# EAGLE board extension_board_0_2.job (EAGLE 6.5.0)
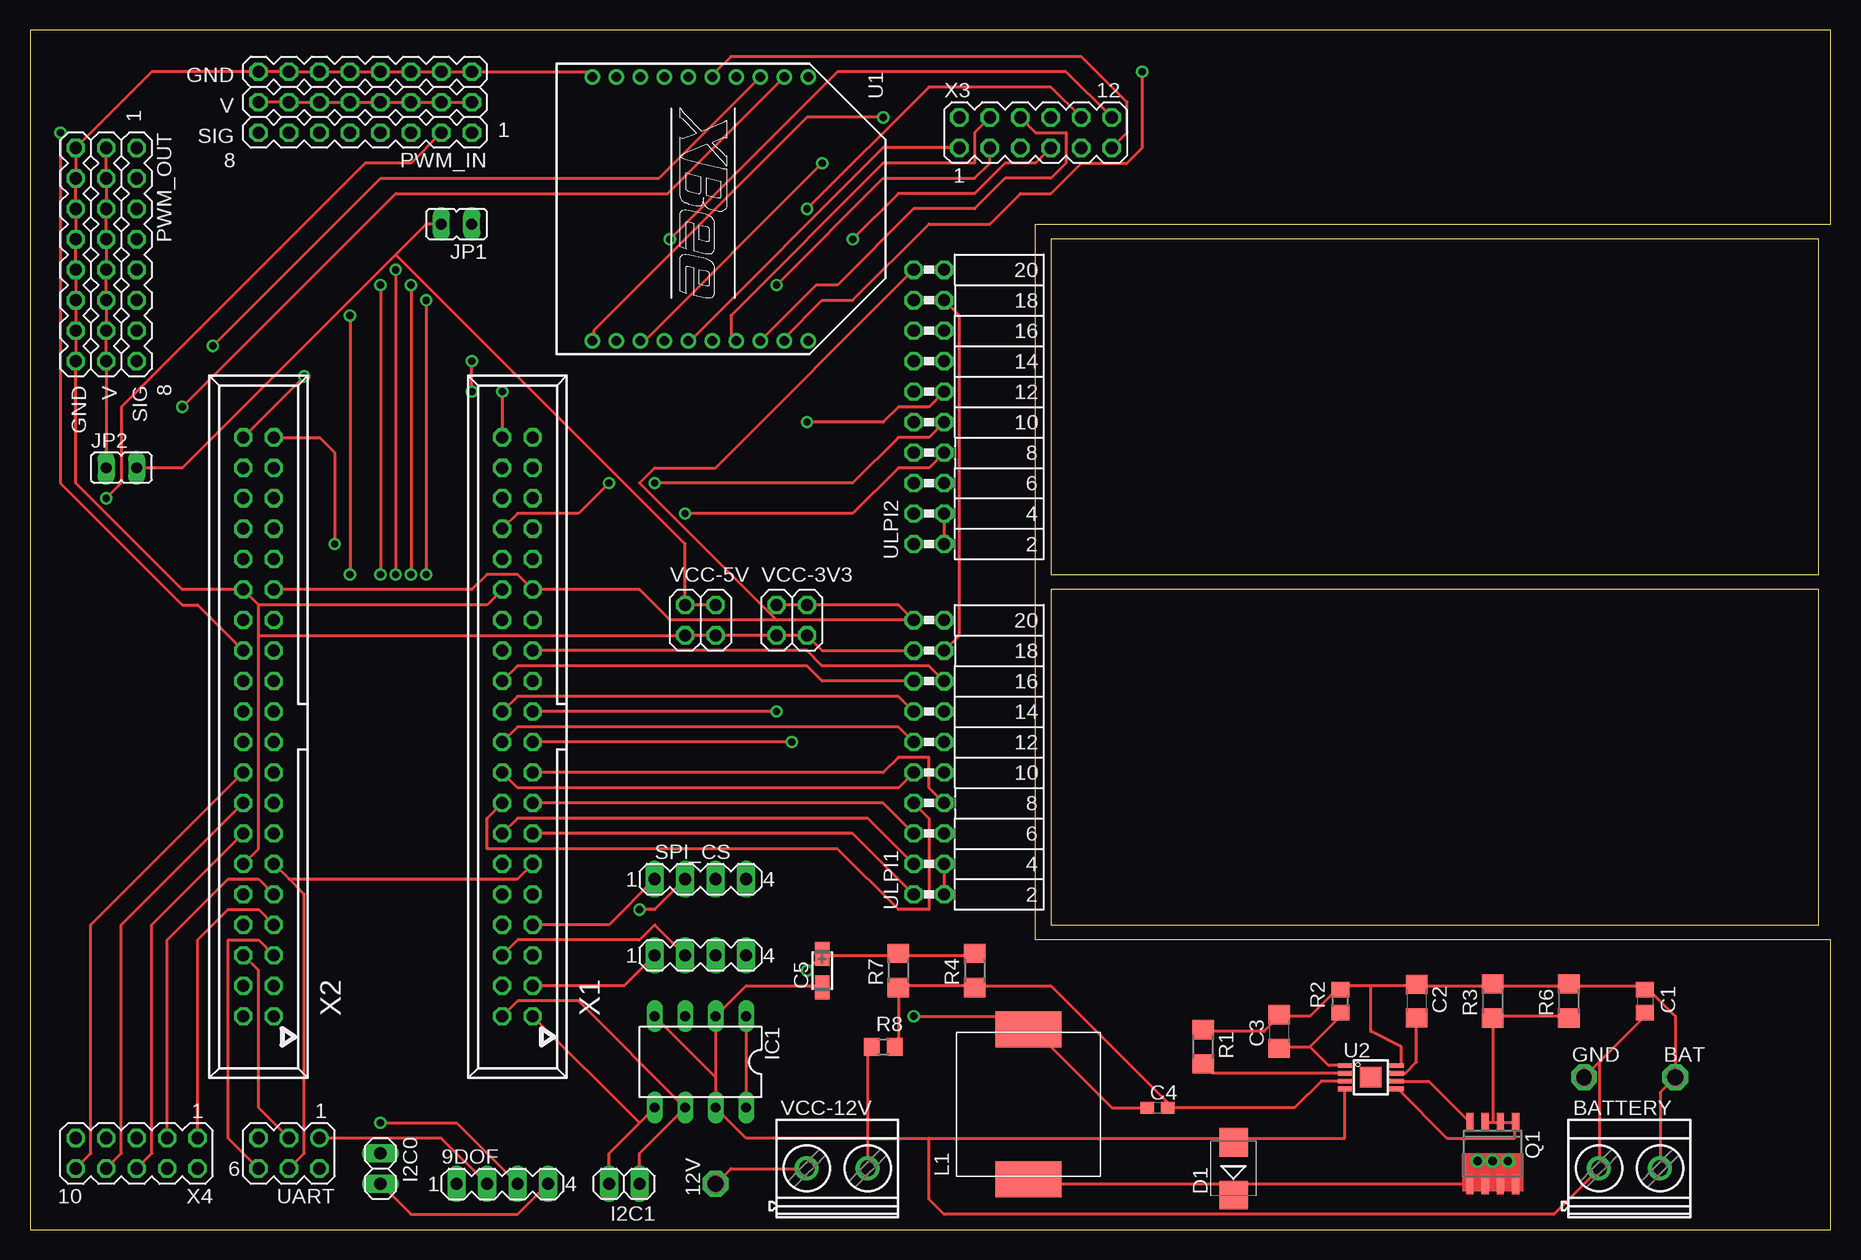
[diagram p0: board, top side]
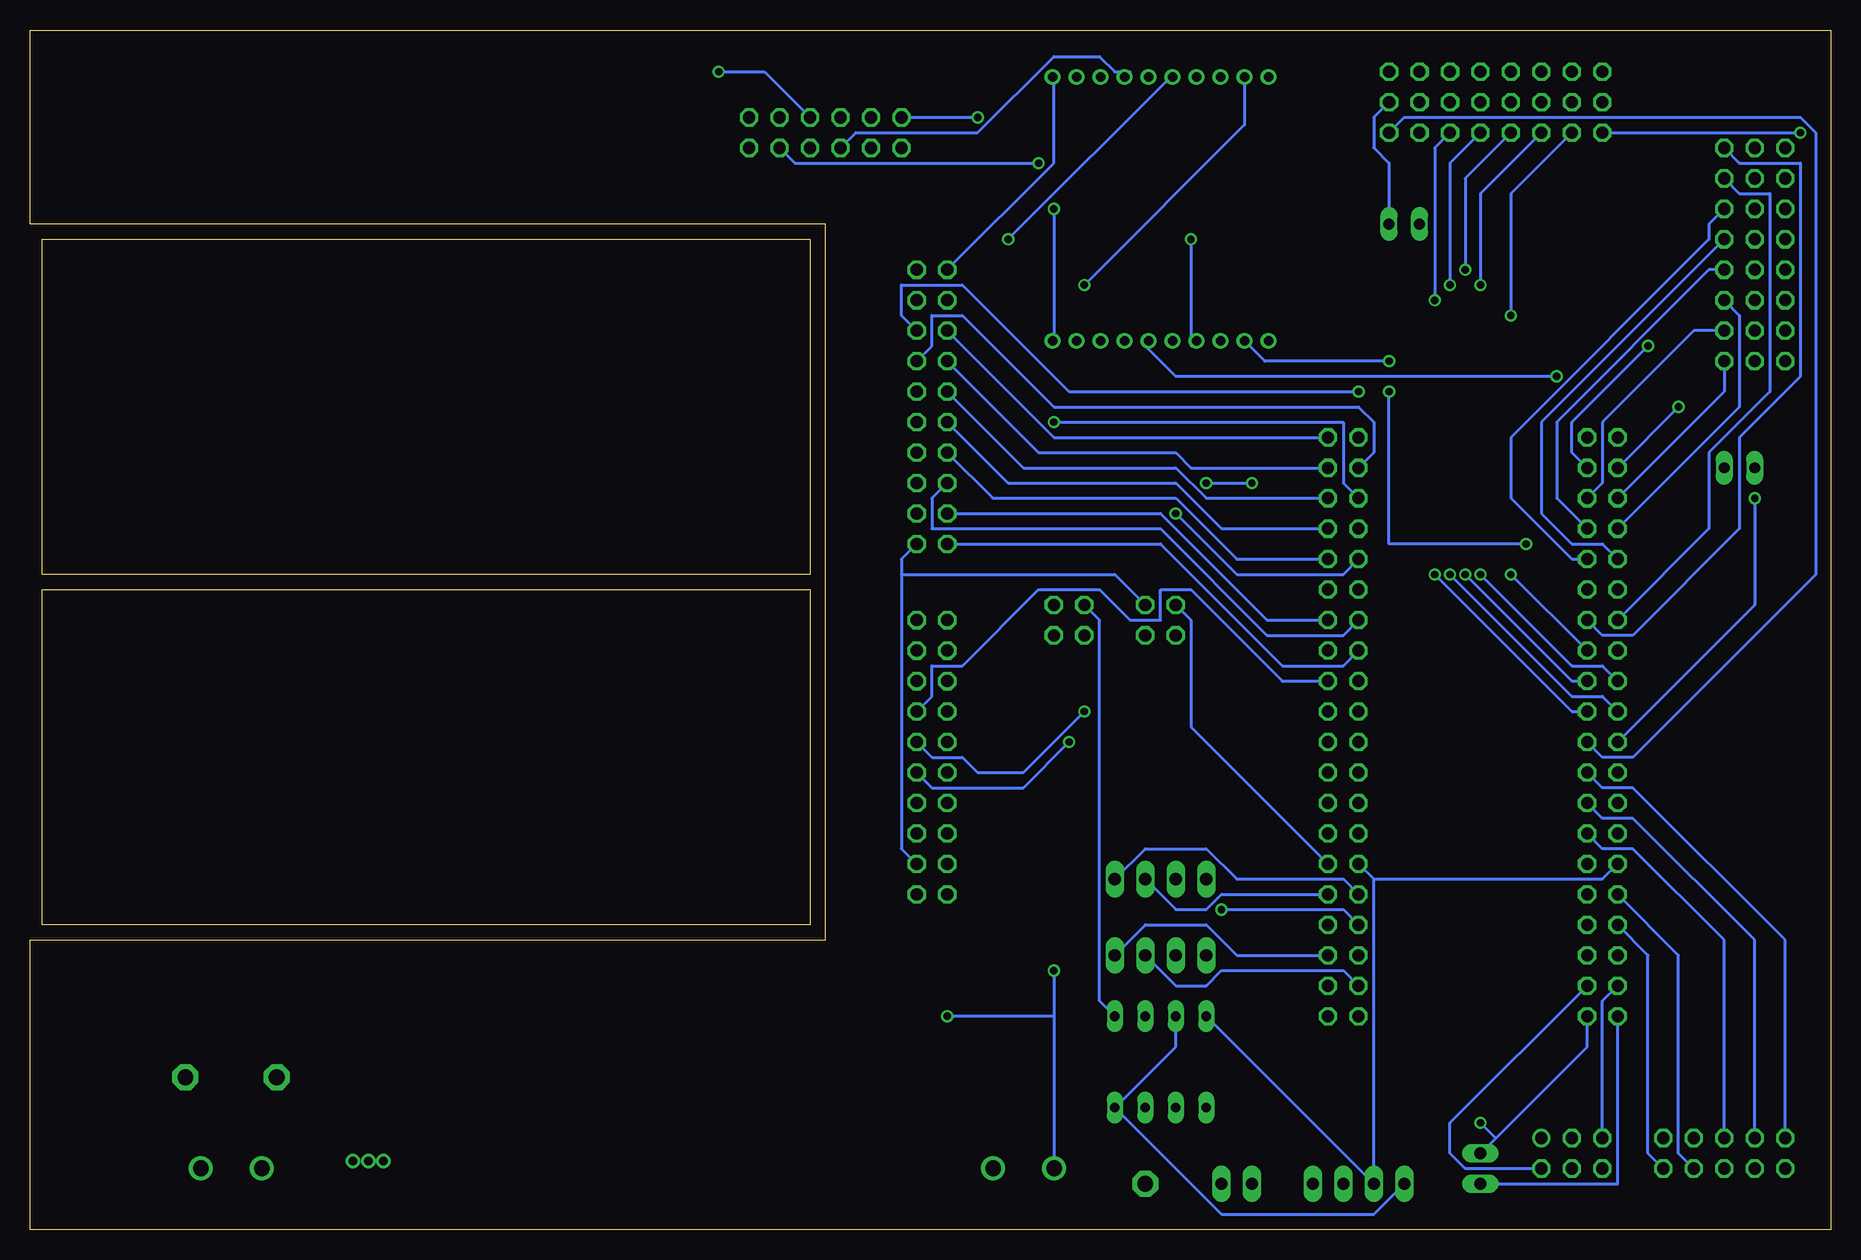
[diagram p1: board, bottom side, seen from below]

Size 150.11 x 100 mm. Coordinates in mm from the lower left corner, seen from the top.
Outline: 0,0 150.11,0 150.11,24.13 83.82,24.13 83.82,83.82 150.11,83.82 150.11,100 0,100 0,0
Copper layers (1*16): Top 0.035mm / dielectric 1.5mm / Bottom 0.035mm
Design rules "default": minimum track width 10mil, minimum drill 24mil, track to track 8mil, track to pad 8mil, pad to pad 8mil, via to via 8mil, smd to smd 8mil, copper to edge 40mil, drill to drill 8mil, minimum pad ring 10mil, minimum via ring 8mil, stop-mask expansion 4mil, vias tented up to drill 0mil, thermal gap 10mil

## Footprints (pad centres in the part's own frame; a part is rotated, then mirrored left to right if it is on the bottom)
MA04-1 = drill 1.016 long: 1 -3.81,0; 2 -1.27,0; 3 1.27,0; 4 3.81,0
P1-13 = drill 1.321 pad 2.159 octagon: TP 0,0
MKDSN1,5/2-5,08 = drill 1.3 pad 2: 1 -2.561,0.025; 2 2.519,0.025
C0805 = smd 1.3 x 1.5: 1 -0.95,0; 2 0.95,0
C1206 = smd 1.6 x 1.8: 1 -1.4,0; 2 1.4,0
C0603 = smd 1.1 x 1: 1 -0.85,0; 2 0.85,0
CT3216 = smd 2 x 1.2: + 1.4,0; - -1.4,0
SMB = smd 2.4 x 2.4: A 2.2,0; C -2.2,0
1X02 = drill 1.016 long: 1 -1.27,0; 2 1.27,0
DIL-08 = drill 0.813 long: 1 -3.81,-3.81; 2 -1.27,-3.81; 3 1.27,-3.81; 4 3.81,-3.81; 5 3.81,3.81; 6 1.27,3.81; 7 -1.27,3.81; 8 -3.81,3.81
JP1 = drill 0.914 long: 1 0,-1.27; 2 0,1.27
INDUKTOR = smd 5.5 x 3: P$1 6,-0.25; P$2 6,12.25
MA08-3 = drill 1.016 octagon: 1-1 -8.89,5.08; 1-2 -6.35,5.08; 1-3 -3.81,5.08; 1-4 -1.27,5.08; 1-5 1.27,5.08; 1-6 3.81,5.08; 1-7 6.35,5.08; 1-8 8.89,5.08; 2-1 -8.89,2.54; 2-2 -6.35,2.54; 2-3 -3.81,2.54; 2-4 -1.27,2.54; 2-5 1.27,2.54; 2-6 3.81,2.54; 2-7 6.35,2.54; 2-8 8.89,2.54; 3-1 -8.89,0; 3-2 -6.35,0; 3-3 -3.81,0; 3-4 -1.27,0; 3-5 1.27,0; 3-6 3.81,0; 3-7 6.35,0; 3-8 8.89,0
SO8-FET = smd 0.6 x 1.6: 1 -1.905,-2.6; 2 -0.635,-2.6; 3 0.635,-2.6; 4 1.905,-2.6; 5 1.905,2.6; 6 0.635,2.6; 7 -0.635,2.6; 8 -1.905,2.6 | drill 0.7: D1 -1.27,0.635; D2 0,0.635; D3 1.27,0.635
R1206 = smd 1.6 x 1.803: 1 -1.422,0; 2 1.422,0
R0805 = smd 1.3 x 1.5: 1 -0.95,0; 2 0.95,0
XBEE = drill 0.8 pad 1.27: 1 -11,9; 2 -11,7; 3 -11,5; 4 -11,3; 5 -11,1; 6 -11,-1; 7 -11,-3; 8 -11,-5; 9 -11,-7; 10 -11,-9; 11 11,-9; 12 11,-7; 13 11,-5; 14 11,-3; 15 11,-1; 16 11,1; 17 11,3; 18 11,5; 19 11,7; 20 11,9
S-PDSO-G08 = smd 0.4 x 1.2: 1 -0.975,-2.157; 2 -0.325,-2.157; 3 0.325,-2.157; 4 0.975,-2.157; 5 0.975,2.157; 6 0.325,2.157; 7 -0.325,2.157; 8 -0.975,2.157 | smd 1.73 x 1.78: TH 0,0
MA03-2 = drill 1.016: 1 -2.54,-1.27 | drill 1.016 octagon: 2 -2.54,1.27; 3 0,-1.27; 4 0,1.27; 5 2.54,-1.27; 6 2.54,1.27
FE10-2W = drill 1.016 octagon: 1 -11.43,1.27; 2 -11.43,-1.27; 3 -8.89,1.27; 4 -8.89,-1.27; 5 -6.35,1.27; 6 -6.35,-1.27; 7 -3.81,1.27; 8 -3.81,-1.27; 9 -1.27,1.27; 10 -1.27,-1.27; 11 1.27,1.27; 12 1.27,-1.27; 13 3.81,1.27; 14 3.81,-1.27; 15 6.35,1.27; 16 6.35,-1.27; 17 8.89,1.27; 18 8.89,-1.27; 19 11.43,1.27; 20 11.43,-1.27
2X02 = drill 1.016 octagon: 1 -1.27,-1.27; 2 -1.27,1.27; 3 1.27,-1.27; 4 1.27,1.27
057-040-1 = drill 1 octagon: 1 -24.13,-1.27; 2 -24.13,1.27; 3 -21.59,-1.27; 4 -21.59,1.27; 5 -19.05,-1.27; 6 -19.05,1.27; 7 -16.51,-1.27; 8 -16.51,1.27; 9 -13.97,-1.27; 10 -13.97,1.27; 11 -11.43,-1.27; 12 -11.43,1.27; 13 -8.89,-1.27; 14 -8.89,1.27; 15 -6.35,-1.27; 16 -6.35,1.27; 17 -3.81,-1.27; 18 -3.81,1.27; 19 -1.27,-1.27; 20 -1.27,1.27; 21 1.27,-1.27; 22 1.27,1.27; 23 3.81,-1.27; 24 3.81,1.27; 25 6.35,-1.27; 26 6.35,1.27; 27 8.89,-1.27; 28 8.89,1.27; 29 11.43,-1.27; 30 11.43,1.27; 31 13.97,-1.27; 32 13.97,1.27; 33 16.51,-1.27; 34 16.51,1.27; 35 19.05,-1.27; 36 19.05,1.27; 37 21.59,-1.27; 38 21.59,1.27; 39 24.13,-1.27; 40 24.13,1.27
MA06-2 = drill 1.016 octagon: 1 -6.35,-1.27; 2 -6.35,1.27; 3 -3.81,-1.27; 4 -3.81,1.27; 5 -1.27,-1.27; 6 -1.27,1.27; 7 1.27,-1.27; 8 1.27,1.27; 9 3.81,-1.27; 10 3.81,1.27; 11 6.35,-1.27; 12 6.35,1.27
MA05-2 = drill 1.016 octagon: 1 -5.08,-1.27; 2 -5.08,1.27; 3 -2.54,-1.27; 4 -2.54,1.27; 5 0,-1.27; 6 0,1.27; 7 2.54,-1.27; 8 2.54,1.27; 9 5.08,-1.27; 10 5.08,1.27

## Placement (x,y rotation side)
9DOF  I2C  [MA04-1]  39.37,3.81 0 top
12V  TPPAD1-13  [P1-13]  57.15,3.81 90 top
BAT  TPPAD1-13  [P1-13]  137.16,12.7 0 top
BATTERY  MKDSN1,5/2-5,08  [MKDSN1,5/2-5,08]  133.35,5.08 0 top
C1  4,7u  [C0805]  134.62,19.05 270 top
C2  470n  [C1206]  115.57,19.05 270 top
C3  1n  [C1206]  104.14,16.51 90 top
C4  7,5 nF  [C0603]  93.98,10.16 0 top
C5  47u  [CT3216]  66.04,21.59 90 top
D1  B340LB  [SMB]  100.33,5.08 90 top
GND  TPPAD1-13  [P1-13]  129.54,12.7 0 top
I2C0  [1X02]  29.21,5.08 270 top
I2C1  [1X02]  49.53,3.81 180 top
IC1  [DIL-08]  55.88,13.97 180 top
JP1  [JP1]  35.56,83.82 90 top
JP2  [JP1]  7.62,63.5 270 top
L1  33u  [INDUKTOR]  77.22,4.42 0 top
PWM_IN  8RX  [MA08-3]  27.94,96.52 180 top
PWM_OUT  8RX  [MA08-3]  3.81,81.28 270 top
Q1  SI4401BDY  [SO8-FET]  121.92,6.35 180 top
R1  274k  [R1206]  97.79,15.24 270 top
R2  1,62k  [R0805]  109.22,19.05 90 top
R3  0,02  [R1206]  121.92,19.05 90 top
R4  20k  [R1206]  78.74,21.59 90 top
R6  0,02  [R1206]  128.27,19.05 90 top
R7  20k  [R1206]  72.39,21.59 90 top
R8  1,15k  [R0805]  71.12,15.24 0 top
SPI  SPI_MAIN  [MA04-1]  55.88,22.86 0 top
SPI_CS  SPI_SS  [MA04-1]  55.88,29.21 0 top
U1  XBEE  [XBEE]  55.88,85.09 270 top
U2  LM5085  [S-PDSO-G08]  111.76,12.7 270 top
UART  UART  [MA03-2]  21.59,6.35 180 top
ULPI1  [FE10-2W]  74.93,39.37 90 top
ULPI2  [FE10-2W]  74.93,68.58 90 top
VCC-3V3  [2X02]  63.5,50.8 0 top
VCC-5V  [2X02]  55.88,50.8 0 top
VCC-12V  MKDSN1,5/2-5,08  [MKDSN1,5/2-5,08]  67.31,5.08 0 top
X1  057-040-1  [057-040-1]  40.64,41.91 90 top
X2  057-040-1  [057-040-1]  19.05,41.91 90 top
X3  [MA06-2]  83.82,91.44 0 top
X4  [MA05-2]  8.89,6.35 180 top

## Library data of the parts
9DOF D1 L1 PWM_IN PWM_OUT SPI SPI_CS U2 UART = multicopter
12V BAT GND = testpad
BATTERY VCC-12V = con-phoenix-508; MPN: MKDSN 1,5/2-5.08; OC_FARNELL: 1792903; OC_NEWARK: 30M2397
C1-C4 = eagle-ltspice; SPICEMODEL: NONE; SPICEPREFIX: C
C5 = resistor
I2C0 I2C1 VCC-3V3 VCC-5V = pinhead
IC1 = solar
JP1 JP2 = jumper
Q1 = probox-parts
R1-R4 R6-R8 = eagle-ltspice; SPICEMODEL: NONE; SPICEPREFIX: R
U1 = maxstream; MPN: XBP24-Z7UIT-004; OC_FARNELL: 1751799; OC_NEWARK: 34R5507
ULPI1 ULPI2 = multicopter; OC_FARNELL: unknown; OC_NEWARK: unknown
X1 X2 = con-panduit; OC_FARNELL: unknown; OC_NEWARK: unknown
X3 X4 = con-lstb; OC_FARNELL: unknown; OC_NEWARK: unknown

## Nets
+3V3: 9DOF.1 IC1.1 IC1.3 IC1.8 U1.1 ULPI1.19 ULPI1.20 ULPI2.19 ULPI2.20 VCC-3V3.2 VCC-3V3.4 X1.29 X2.29
+5V: JP1.2 JP2.2 UART.4 ULPI1.2 ULPI1.4 ULPI2.2 ULPI2.4 VCC-5V.2 VCC-5V.4 X1.11 X2.11
+12V: 12V.TP C4.1 C5.+ L1.P$2 R4.2 R7.2 VCC-12V.1
GND: 9DOF.2 BATTERY.1 C1.2 C5.- D1.A GND.TP IC1.2 IC1.4 IC1.7 PWM_IN.3-1 PWM_IN.3-2 PWM_IN.3-3 PWM_IN.3-4 PWM_IN.3-5 PWM_IN.3-6 PWM_IN.3-7 PWM_IN.3-8 PWM_OUT.3-1 PWM_OUT.3-2 PWM_OUT.3-3 PWM_OUT.3-4 PWM_OUT.3-5 PWM_OUT.3-6 PWM_OUT.3-7 PWM_OUT.3-8 R8.1 U1.10 U2.4 UART.1 ULPI1.17 ULPI1.18 ULPI2.17 ULPI2.18 VCC-3V3.1 VCC-3V3.3 VCC-5V.1 VCC-5V.3 VCC-12V.2 X1.12 X1.30 X2.12 X2.30
GPIO0: X2.7 X4.1
GPIO1: X2.8 X4.2
GPIO2: X2.9 X4.3
GPIO3: X2.10 X4.4
GPIO4: X2.13 X4.5
GPIO5: X2.14 X4.6
GPIO6: X2.15 X4.7
GPIO7: X2.16 X4.8
GPIO8: X2.17 X4.9
GPIO9: X2.18 X4.10
I2C-0-SCL: 9DOF.4 I2C0.2 X2.2
I2C-0-SDA: 9DOF.3 I2C0.1 X2.1
I2C-1-SCL: I2C1.1 IC1.6 X1.2
I2C-1-SDA: I2C1.2 IC1.5 X1.1
N$3: R1.2 U2.2
N$4: C2.2 U2.7
N$5: C3.1 R2.1 U2.1
N$7: Q1.1 Q1.2 Q1.3 R3.1 R6.1 U2.5
N$8: C4.2 R4.1 R7.1 R8.2 U2.3
N$9: Q1.4 U2.6
N$10: D1.C L1.P$1 Q1.5 Q1.6 Q1.7 Q1.8 Q1.D1 Q1.D2 Q1.D3
N$11: JP1.1 PWM_IN.2-1 PWM_IN.2-2 PWM_IN.2-3 PWM_IN.2-4 PWM_IN.2-5 PWM_IN.2-6 PWM_IN.2-7 PWM_IN.2-8
N$12: JP2.1 PWM_OUT.2-1 PWM_OUT.2-2 PWM_OUT.2-3 PWM_OUT.2-4 PWM_OUT.2-5 PWM_OUT.2-6 PWM_OUT.2-7 PWM_OUT.2-8
N$23: U1.5 X3.11
N$24: U1.14 X3.12
N$25: U1.20 X3.10
N$26: U1.19 X3.8
N$27: U1.18 X3.6
N$28: U1.17 X3.4
N$29: U1.11 X3.2
N$30: U1.15 X3.1
N$31: U1.9 X3.3
N$32: U1.4 X3.5
N$33: U1.6 X3.7
N$34: U1.13 X3.9
PWM_IN1: PWM_IN.1-1 X2.19
PWM_IN2: PWM_IN.1-2 X2.20
PWM_IN3: PWM_IN.1-3 X2.21
PWM_IN4: PWM_IN.1-4 X2.22
PWM_IN5: PWM_IN.1-5 X2.23
PWM_IN6: PWM_IN.1-6 X2.24
PWM_IN7: PWM_IN.1-7 X2.25
PWM_IN8: PWM_IN.1-8 X2.26
PWM_OUT1: PWM_OUT.1-1 X2.27
PWM_OUT2: PWM_OUT.1-2 X2.28
PWM_OUT3: PWM_OUT.1-3 X2.31
PWM_OUT4: PWM_OUT.1-4 X2.32
PWM_OUT5: PWM_OUT.1-5 X2.33
PWM_OUT6: PWM_OUT.1-6 X2.34
PWM_OUT7: PWM_OUT.1-7 X2.35
PWM_OUT8: PWM_OUT.1-8 X2.36
SPI_CLK: SPI.1 X1.3
SPI_MISO: SPI.4 X1.5
SPI_MOSI: SPI.3 X1.4
SPI_SS: SPI.2 X1.6
SPI_SS0: SPI_CS.1 X1.7
SPI_SS1: SPI_CS.2 X1.8
SPI_SS2: SPI_CS.3 X1.9
SPI_SS3: SPI_CS.4 X1.10
UART_CTS: UART.3 X2.6
UART_RTS: UART.6 X2.5
UART_RX: UART.2 X2.3
UART_TX: UART.5 X2.4
ULPI1_CLK: ULPI1.10 X1.19
ULPI1_D0: ULPI1.1 X1.13
ULPI1_D1: ULPI1.3 X1.14
ULPI1_D2: ULPI1.5 X1.15
ULPI1_D3: ULPI1.7 X1.16
ULPI1_D4: ULPI1.9 X1.18
ULPI1_D5: ULPI1.11 X1.20
ULPI1_D6: ULPI1.13 X1.22
ULPI1_D7: ULPI1.15 X1.24
ULPI1_DIR: ULPI1.12 X1.21
ULPI1_NXT: ULPI1.14 X1.23
ULPI1_RST: ULPI1.8 X1.17
ULPI1_STP: ULPI1.16 X1.25
ULPI2_CLK: ULPI2.10 X1.34
ULPI2_D0: ULPI2.1 X1.26
ULPI2_D1: ULPI2.3 X1.27
ULPI2_D2: ULPI2.5 X1.28
ULPI2_D3: ULPI2.7 X1.31
ULPI2_D4: ULPI2.9 X1.33
ULPI2_D5: ULPI2.11 X1.35
ULPI2_D6: ULPI2.13 X1.37
ULPI2_D7: ULPI2.15 X1.39
ULPI2_DIR: ULPI2.12 X1.36
ULPI2_NXT: ULPI2.14 X1.38
ULPI2_RST: ULPI2.8 X1.32
ULPI2_STP: ULPI2.16 X1.40
VCC-BAT: BAT.TP BATTERY.2 C1.1 C2.1 C3.2 R1.1 R2.2 R3.2 R6.2 U2.8
XBEE-CTS: U1.12 X2.39
XBEE-RTS: U1.16 X2.40
XBEE-RX: U1.2 X2.38
XBEE-TX: U1.3 X2.37

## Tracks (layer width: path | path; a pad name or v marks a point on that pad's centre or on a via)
+3V3
  Top 0.254: ULPI2.20 ULPI2.19 57.15,63.5 52.07,63.5 50.8,62.23 62.23,50.8 | X2.29 36.83,53.34 38.1,54.61 40.64,54.61 X1.29 50.8,53.34 53.34,50.8 62.23,50.8 | VCC-3V3.2 VCC-3V3.4 72.39,52.07 ULPI1.19 | ULPI1.20 ULPI1.19 | IC1.1 IC1.8 | ULPI1.19 62.23,50.8
  Bottom 0.254: ULPI2.19 64.77,88.9 64.77,96.52 U1.1 | IC1.3 54.61,15.24 IC1.8 50.8,1.27 38.1,1.27 9DOF.1 | VCC-3V3.2 60.96,50.8 60.96,19.05 IC1.1
+5V
  Top 0.254: 21.59,29.21 22.86,27.94 22.86,6.35 UART.4 | 21.59,29.21 X2.11 | X1.11 40.64,29.21 21.59,29.21 | JP2.2 12.7,63.5 30.48,81.28 | 30.48,81.28 33.02,83.82 JP1.2 | VCC-5V.4 VCC-5V.2 54.61,57.15 30.48,81.28 | ULPI1.4 ULPI1.2 | ULPI2.4 ULPI2.2
  Bottom 0.254: ULPI1.4 77.47,31.75 77.47,54.61 | 77.47,54.61 77.47,55.88 ULPI2.2 | VCC-5V.4 59.69,54.61 77.47,54.61 | X1.11 53.34,41.91 53.34,50.8 VCC-5V.2
+12V  (via drill 0.61)
  Top 0.254: 12V.TP 58.42,5.08 64.77,5.08 VCC-12V.1 | C4.1 90.17,10.16 83.82,16.51 L1.P$2 82.55,17.78 v73.66,17.78 | 66.04,22.86 72.39,22.86 | 72.39,22.86 78.74,22.86 R4.2 | 72.39,22.86 R7.2 | 66.04,22.86 v64.77,21.59 | 66.04,22.86 C5.+
  Bottom 0.254: v64.77,21.59 64.77,17.78 | 64.77,17.78 64.77,5.08 VCC-12V.1 | 64.77,17.78 v73.66,17.78
GND
  Top 0.254: U1.10 46.99,96.52 PWM_IN.3-1 PWM_IN.3-2 PWM_IN.3-3 PWM_IN.3-4 PWM_IN.3-5 PWM_IN.3-6 PWM_IN.3-7 PWM_IN.3-8 10.16,96.52 PWM_OUT.3-1 PWM_OUT.3-2 PWM_OUT.3-3 PWM_OUT.3-4 PWM_OUT.3-5 PWM_OUT.3-6 PWM_OUT.3-7 PWM_OUT.3-8 3.81,62.23 12.7,53.34 X2.30 19.05,52.07 | ULPI2.17 ULPI2.18 77.47,76.2 77.47,49.53 ULPI1.18 ULPI1.17 66.04,48.26 VCC-3V3.3 VCC-3V3.1 VCC-5V.3 VCC-5V.1 19.05,49.53 | 19.05,52.07 38.1,52.07 X1.30 | 57.15,12.7 IC1.2 59.69,20.32 66.04,20.32 C5.- | 57.15,12.7 IC1.7 59.69,7.62 69.85,7.62 | 57.15,12.7 IC1.4 | UART.1 34.29,7.62 9DOF.2 | 19.05,49.53 19.05,31.75 X2.12 | 19.05,49.53 19.05,52.07 | GND.TP 130.81,13.97 | 130.81,13.97 134.62,17.78 C1.2 | 130.81,13.97 130.81,5.08 | 130.81,5.08 BATTERY.1 | 69.85,7.62 69.85,5.08 VCC-12V.2 | 69.85,7.62 69.85,15.24 R8.1 | 69.85,7.62 74.93,7.62 | 74.93,7.62 100.33,7.62 | 100.33,7.62 D1.A | 100.33,7.62 109.6,7.62 U2.4 | 130.81,5.08 127,1.27 76.2,1.27 74.93,2.54 74.93,7.62
  Bottom 0.254: X2.12 19.05,29.21 38.1,29.21 | X1.12 38.1,29.21 | IC1.4 9DOF.2 38.1,29.21
GPIO0
  Top 0.254: X2.7 19.05,26.67 16.51,26.67 13.97,24.13 X4.1
GPIO1
  Bottom 0.254: X2.8 15.24,22.86 15.24,6.35 X4.2
GPIO2
  Top 0.254: X2.9 19.05,29.21 16.51,29.21 11.43,24.13 X4.3
GPIO3
  Bottom 0.254: X2.10 12.7,22.86 12.7,6.35 X4.4
GPIO4
  Bottom 0.254: X2.13 19.05,31.75 16.51,31.75 8.89,24.13 X4.5
GPIO5
  Top 0.254: X2.14 10.16,25.4 10.16,6.35 X4.6
GPIO6
  Bottom 0.254: X2.15 19.05,34.29 16.51,34.29 6.35,24.13 X4.7
GPIO7
  Top 0.254: X2.16 7.62,25.4 7.62,6.35 X4.8
GPIO8
  Bottom 0.254: X2.17 19.05,36.83 16.51,36.83 3.81,24.13 X4.9
GPIO9
  Top 0.254: X2.18 5.08,25.4 5.08,6.35 X4.10
I2C-0-SCL
  Top 0.254: 9DOF.4 40.64,1.27 31.75,1.27 I2C0.2
  Bottom 0.254: X2.2 17.78,3.81 I2C0.2
I2C-0-SDA  (via drill 0.61)
  Top 0.254: 9DOF.3 35.56,8.89 v29.21,8.89
  Bottom 0.254: X2.1 20.32,15.24 27.94,7.62 | I2C0.1 27.94,7.62 | 27.94,7.62 v29.21,8.89
I2C-1-SCL
  Top 0.254: I2C1.1 50.8,6.35 IC1.6 45.72,19.05 40.64,19.05 X1.2
I2C-1-SDA
  Top 0.254: 50.8,8.89 48.26,6.35 I2C1.2 | 50.8,8.89 IC1.5 | 50.8,8.89 X1.1
N$3
  Top 0.254: U2.2 98.58,13.03 R1.2
N$4
  Top 0.254: U2.7 114.62,13.03 115.57,13.97 C2.2
N$5
  Top 0.254: 106.68,15.24 109.22,17.78 R2.1 | 106.68,15.24 104.14,15.24 C3.1 | U2.1 108.25,13.68 106.68,15.24
N$7
  Top 0.254: R6.1 128.27,17.78 121.92,17.78 R3.1 121.92,8.95 | Q1.3 121.92,8.95 | 121.92,8.95 Q1.2 Q1.1 123.77,7.62 118.11,7.62 114,11.72 U2.5
N$8
  Top 0.254: R8.2 72.39,15.24 R7.1 72.39,20.32 78.74,20.32 | 78.74,20.32 85.09,20.32 95.25,10.16 C4.2 105.41,10.16 107.62,12.38 U2.3 | 78.74,20.32 R4.1
N$9
  Top 0.254: U2.6 116.59,12.38 Q1.4
N$10
  Top 0.254: 100.33,3.81 83.82,3.81 L1.P$1 | 100.33,3.81 D1.C | 100.33,3.81 119.95,3.81 Q1.5 Q1.6 Q1.7 | Q1.7 Q1.8 | Q1.7 123.19,3.75 Q1.D1 Q1.D2 Q1.D3
N$11
  Top 0.254: PWM_IN.2-8 PWM_IN.2-7 PWM_IN.2-6 PWM_IN.2-5 PWM_IN.2-4 PWM_IN.2-3 PWM_IN.2-2 PWM_IN.2-1
  Bottom 0.254: JP1.1 36.83,88.9 38.1,90.17 38.1,92.71 PWM_IN.2-1
N$12
  Top 0.254: PWM_OUT.2-1 PWM_OUT.2-2 PWM_OUT.2-3 PWM_OUT.2-4 PWM_OUT.2-5 PWM_OUT.2-6 PWM_OUT.2-7 PWM_OUT.2-8 JP2.1
N$23
  Top 0.254: X3.11 91.44,91.44 91.44,93.98 87.63,97.79 58.42,97.79 57.15,96.52 U1.5
N$24  (via drill 0.61)
  Top 0.254: v53.34,82.55 67.31,96.52 86.36,96.52 X3.12
  Bottom 0.254: v53.34,82.55 53.34,73.66 U1.14
N$25  (via drill 0.61)
  Top 0.254: v64.77,85.09 74.93,95.25 85.09,95.25 X3.10
  Bottom 0.254: v64.77,85.09 64.77,73.66 U1.20
N$26  (via drill 0.61)
  Top 0.254: U1.19 62.88,74.31 66.04,77.47 68.58,77.47 74.93,83.82 80.01,83.82 82.55,86.36 85.09,86.36 87.63,88.9 91.44,88.9 92.71,90.17 v92.71,96.52
  Bottom 0.254: v92.71,96.52 88.9,96.52 X3.8
N$27
  Top 0.254: X3.6 83.82,91.44 86.36,91.44 86.36,88.9 85.09,87.63 81.28,87.63 78.74,85.09 73.66,85.09 67.31,78.74 65.53,78.74 U1.18
N$28
  Top 0.254: X3.4 78.74,91.44 78.74,88.9 71.12,88.9 58.42,76.2 58.42,73.66 U1.17
N$29  (via drill 0.61)
  Top 0.254: v71.12,92.71 64.77,92.71 46.99,74.93 46.99,73.66 U1.11
  Bottom 0.254: X3.2 v71.12,92.71
N$30
  Top 0.254: X3.1 71.12,90.17 54.61,73.66 U1.15
N$31  (via drill 0.61)
  Top 0.254: v62.23,78.74 71.12,87.63 78.74,87.63 80.01,88.9 X3.3
  Bottom 0.254: U1.9 48.88,92.09 v62.23,78.74
N$32
  Bottom 0.254: X3.5 81.28,91.44 71.12,91.44 64.77,97.79 60.96,97.79 59.69,96.52 58.42,96.52 U1.4
N$33  (via drill 0.61)
  Top 0.254: v68.58,82.55 72.39,86.36 78.74,86.36 81.28,88.9 83.82,88.9 X3.7
  Bottom 0.254: v68.58,82.55 54.61,96.52 U1.6
N$34  (via drill 0.61)
  Top 0.254: v66.04,88.9 50.8,73.66 U1.13
  Bottom 0.254: v66.04,88.9 86.36,88.9 X3.9
PWM_IN1
  Bottom 0.254: X2.19 19.05,39.37 16.51,39.37 1.27,54.61 1.27,91.44 2.54,92.71 35.56,92.71 PWM_IN.1-1
PWM_IN2  (via drill 0.61)
  Top 0.254: v6.35,60.96 7.62,62.23 7.62,68.58 27.94,88.9 31.75,88.9 PWM_IN.1-2
  Bottom 0.254: X2.20 6.35,52.07 v6.35,60.96
PWM_IN3  (via drill 0.61)
  Top 0.254: v33.02,77.47 v33.02,54.61
  Bottom 0.254: X2.21 21.59,43.18 v33.02,54.61 | v33.02,77.47 33.02,90.17 PWM_IN.1-3
PWM_IN4  (via drill 0.61)
  Top 0.254: v31.75,78.74 v31.75,54.61
  Bottom 0.254: X2.22 19.05,44.45 21.59,44.45 v31.75,54.61 | v31.75,78.74 31.75,88.9 PWM_IN.1-4
PWM_IN5  (via drill 0.61)
  Top 0.254: v30.48,80.01 v30.48,54.61
  Bottom 0.254: X2.23 21.59,45.72 v30.48,54.61 | v30.48,80.01 30.48,87.63 PWM_IN.1-5
PWM_IN6  (via drill 0.61)
  Top 0.254: v29.21,78.74 v29.21,54.61
  Bottom 0.254: X2.24 19.05,46.99 21.59,46.99 v29.21,54.61 | v29.21,78.74 29.21,86.36 PWM_IN.1-6
PWM_IN7  (via drill 0.61)
  Top 0.254: v26.67,76.2 v26.67,54.61
  Bottom 0.254: v26.67,54.61 X2.25 | v26.67,76.2 26.67,86.36 PWM_IN.1-7
PWM_IN8  (via drill 0.61)
  Top 0.254: X2.26 13.97,52.07 12.7,52.07 2.54,62.23 v2.54,91.44
  Bottom 0.254: PWM_IN.1-8 v2.54,91.44
PWM_OUT1
  Bottom 0.254: X2.27 19.05,49.53 16.51,49.53 7.62,58.42 7.62,66.04 2.54,71.12 2.54,88.9 7.62,88.9 PWM_OUT.1-1
PWM_OUT2
  Bottom 0.254: X2.28 10.16,58.42 10.16,64.77 5.08,69.85 5.08,86.36 7.62,86.36 PWM_OUT.1-2
PWM_OUT3
  Bottom 0.254: X2.31 21.59,55.88 26.67,60.96 26.67,66.04 10.16,82.55 10.16,83.82 PWM_OUT.1-3
PWM_OUT4
  Bottom 0.254: X2.32 19.05,57.15 21.59,57.15 24.13,59.69 24.13,67.31 PWM_OUT.1-4
PWM_OUT5
  Bottom 0.254: X2.33 22.86,60.96 22.86,67.31 10.16,80.01 PWM_OUT.1-5
PWM_OUT6
  Bottom 0.254: X2.34 7.62,68.58 7.62,76.2 PWM_OUT.1-6
PWM_OUT7
  Bottom 0.254: X2.35 19.05,62.23 19.05,67.31 11.43,74.93 PWM_OUT.1-7
PWM_OUT8
  Bottom 0.254: X2.36 8.89,69.85 PWM_OUT.1-8
SPI_CLK
  Top 0.254: X1.3 49.53,20.32 SPI.1
SPI_MISO
  Bottom 0.254: X1.5 49.53,22.86 52.07,25.4 57.15,25.4 SPI.4
SPI_MOSI
  Bottom 0.254: X1.4 40.64,21.59 50.8,21.59 52.07,20.32 54.61,20.32 SPI.3
SPI_SS
  Top 0.254: X1.6 40.64,24.13 50.8,24.13 52.07,25.4 SPI.2
SPI_SS0
  Top 0.254: X1.7 48.26,25.4 SPI_CS.1
SPI_SS1  (via drill 0.61)
  Top 0.254: v50.8,26.67 52.07,26.67 SPI_CS.2
  Bottom 0.254: X1.8 40.64,26.67 v50.8,26.67
SPI_SS2
  Bottom 0.254: X1.9 50.8,27.94 52.07,26.67 54.61,26.67 SPI_CS.3
SPI_SS3
  Bottom 0.254: X1.10 40.64,29.21 49.53,29.21 52.07,31.75 57.15,31.75 SPI_CS.4
UART_CTS
  Top 0.254: X2.6 19.05,21.59 19.05,10.16 UART.3
UART_RTS
  Top 0.254: X2.5 19.05,24.13 16.51,24.13 16.51,7.62 UART.6
UART_RX
  Bottom 0.254: X2.3 31.75,8.89 31.75,6.35 30.48,5.08 UART.2
UART_TX
  Bottom 0.254: X2.4 19.05,19.05 UART.5
ULPI1_CLK  (via drill 0.61)
  Top 0.254: v63.5,40.64 X1.19
  Bottom 0.254: v63.5,40.64 67.31,36.83 74.93,36.83 ULPI1.10
ULPI1_D0
  Top 0.254: X1.13 68.58,33.02 ULPI1.1
ULPI1_D1
  Top 0.254: X1.14 40.64,34.29 69.85,34.29 ULPI1.3
ULPI1_D2
  Top 0.254: X1.15 71.12,35.56 ULPI1.5
ULPI1_D3
  Top 0.254: X1.16 38.1,34.29 38.1,31.75 67.31,31.75 72.39,26.67 74.93,26.67 74.93,34.29 ULPI1.7
ULPI1_D4
  Top 0.254: X1.18 40.64,36.83 72.39,36.83 ULPI1.9
ULPI1_D5
  Top 0.254: X1.20 40.64,41.91 72.39,41.91 ULPI1.11
ULPI1_D6
  Top 0.254: X1.22 40.64,44.45 72.39,44.45 ULPI1.13
ULPI1_D7
  Top 0.254: X1.24 40.64,46.99 64.77,46.99 66.04,45.72 ULPI1.15
ULPI1_DIR  (via drill 0.61)
  Top 0.254: v62.23,43.18 X1.21
  Bottom 0.254: v62.23,43.18 67.31,38.1 71.12,38.1 72.39,39.37 74.93,39.37 ULPI1.12
ULPI1_NXT
  Bottom 0.254: X1.23 45.72,45.72 53.34,53.34 55.88,53.34 55.88,50.8 58.42,50.8 60.96,53.34 66.04,53.34 72.39,46.99 74.93,46.99 74.93,44.45 ULPI1.14
ULPI1_RST
  Top 0.254: X1.17 71.12,38.1 72.39,39.37 74.93,39.37 74.93,36.83 ULPI1.8
ULPI1_STP
  Top 0.254: X1.25 64.77,48.26 66.04,46.99 74.93,46.99 ULPI1.16
ULPI2_CLK  (via drill 0.61)
  Top 0.254: X1.34 40.64,59.69 45.72,59.69 v48.26,62.23 | v52.07,62.23 68.58,62.23 72.39,66.04 74.93,66.04 ULPI2.10
  Bottom 0.254: v52.07,62.23 v48.26,62.23
ULPI2_D0
  Bottom 0.254: X1.26 40.64,46.99 45.72,46.99 55.88,57.15 ULPI2.1
ULPI2_D1
  Bottom 0.254: X1.27 46.99,50.8 55.88,59.69 ULPI2.3
ULPI2_D2
  Bottom 0.254: X1.28 40.64,49.53 46.99,49.53 55.88,58.42 74.93,58.42 74.93,60.96 ULPI2.5
ULPI2_D3
  Bottom 0.254: X1.31 49.53,55.88 54.61,60.96 69.85,60.96 ULPI2.7
ULPI2_D4
  Bottom 0.254: X1.33 50.8,58.42 54.61,62.23 68.58,62.23 ULPI2.9
ULPI2_D5
  Bottom 0.254: X1.35 52.07,60.96 54.61,63.5 67.31,63.5 ULPI2.11
ULPI2_D6
  Bottom 0.254: X1.37 53.34,63.5 54.61,64.77 66.04,64.77 ULPI2.13
ULPI2_D7
  Bottom 0.254: X1.39 64.77,66.04 ULPI2.15
ULPI2_DIR  (via drill 0.61)
  Top 0.254: v64.77,67.31 71.12,67.31 72.39,68.58 74.93,68.58 ULPI2.12
  Bottom 0.254: X1.36 40.64,62.23 40.64,67.31 v64.77,67.31
ULPI2_NXT
  Bottom 0.254: X1.38 38.1,64.77 38.1,67.31 39.37,68.58 64.77,68.58 72.39,76.2 74.93,76.2 74.93,73.66 ULPI2.14
ULPI2_RST  (via drill 0.61)
  Top 0.254: v54.61,59.69 68.58,59.69 72.39,63.5 74.93,63.5 ULPI2.8
  Bottom 0.254: X1.32 40.64,54.61 49.53,54.61 v54.61,59.69
ULPI2_STP  (via drill 0.61)
  Top 0.254: v39.37,69.85 X1.40
  Bottom 0.254: v39.37,69.85 63.5,69.85 72.39,78.74 77.47,78.74 77.47,76.2 ULPI2.16
VCC-BAT
  Top 0.254: BATTERY.2 135.89,5.08 135.89,11.43 BAT.TP 137.16,17.78 134.62,20.32 | 128.27,20.32 134.62,20.32 | 115.57,20.32 111.76,20.32 | 111.76,20.32 109.22,20.32 | 104.14,17.78 106.68,17.78 109.22,20.32 | 109.22,20.32 R2.2 | 104.14,17.78 102.87,16.51 97.79,16.51 R1.1 | 104.14,17.78 C3.2 | 115.57,20.32 121.92,20.32 | 115.57,20.32 C2.1 | 121.92,20.32 128.27,20.32 | 128.27,20.32 R6.2 | 121.92,20.32 R3.2 | 134.62,20.32 C1.1 | U2.8 114.3,13.68 114.3,15.24 111.76,16.51 111.76,20.32
XBEE-CTS  (via drill 0.61)
  Top 0.254: X2.39 24.13,66.04 25.4,64.77 v25.4,57.15 | v36.83,69.85 v36.83,72.39
  Bottom 0.254: v25.4,57.15 36.83,57.15 v36.83,69.85 | v36.83,72.39 47.18,72.39 U1.12
XBEE-RTS  (via drill 0.61)
  Top 0.254: X2.40 v22.86,71.12
  Bottom 0.254: v22.86,71.12 54.61,71.12 57.15,73.66 U1.16
XBEE-RX  (via drill 0.61)
  Top 0.254: v12.7,68.58 30.48,86.36 53.15,86.36 U1.2
  Bottom 0.254: X2.38 v12.7,68.58
XBEE-TX  (via drill 0.61)
  Top 0.254: v15.24,73.66 29.21,87.63 52.42,87.63 U1.3
  Bottom 0.254: v15.24,73.66 21.59,67.31 21.59,64.77 X2.37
